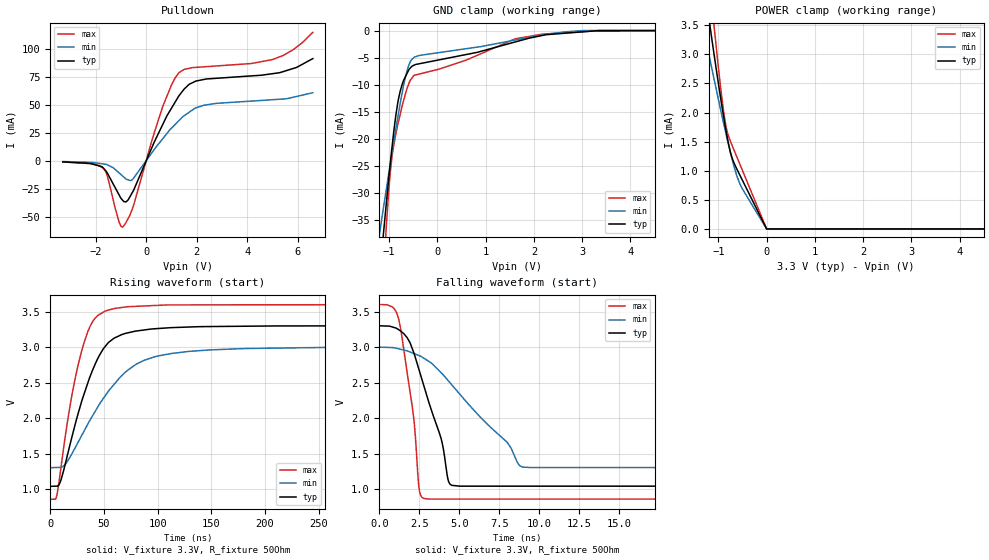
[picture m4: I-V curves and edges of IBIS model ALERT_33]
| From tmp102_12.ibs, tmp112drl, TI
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|   ALERT_33   3.3V digital open-drain Model
[Model] ALERT_33
Model_type   Open_drain
| Signals   ALERT(3)
Polarity   Non-Inverting
Enable   Active-Low
Vmeas = 1.65
Vref = 1.65
Cref = 15pF
Rref = 50
|   typ   min   max
|   (nom PVT)   (Fast PVT)   (slow PVT)
|   output low
|C_comp   1.4655810e-10   5.2129330e-11  1.1989730e-10
| Where   nom PVT is  Nominal Process, 3.3V, -40C
|   Fast PVT is Strong Process, 3.6V, 125C
|   Slow PVT is Weak Process, 3.0V, 27C
|   output high
C_comp   1.8565580e-12  1.4984630e-12  2.4264050e-12
| Where   nom PVT is  Nominal Process, 1.5V, 27C
|   Fast PVT is Strong Process, 1.6V, -40C
|   Slow PVT is Weak Process, 1.4V, 125C
[Voltage Range]   3.3   3   3.6
[Temperature Range]   27   125   -40
|Ambient Temperature   27   125   -40
[Pullup Reference]   3.3   3   3.6
[Pulldown Reference]   0   0   0
[Power Clamp Reference]   3.3   3   3.6
[GND Clamp Reference]   0   0   0
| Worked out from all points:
|   slope of the pulldown table from 0 to 0.495 V, typ, clamps not added: 19.8 ohm
|   POWER clamp passes 1 mA (typ) near -0.60 V on its own axis
|   falling waveform, V_fixture 3.3V, R_fixture 50Ohm: 20-80 % time 1.8ns typ, 4.29ns min, 878ps max; typ from 3.3 V to 1.04 V
|   rising waveform, V_fixture 3.3V, R_fixture 50Ohm: 20-80 % time 28.3ns typ, 45.8ns min, 20.4ns max; typ from 1.04 V to 3.3 V
[Pulldown]
|   Voltage   I(typ)   I(min)   I(max)
-3.3V     -1.098mA   -766.7uA   -1.108mA
-1.681V   -7.048mA   -2.977mA   -7.001mA
-1.529V   -11.45mA   -3.762mA   -14.26mA
-1.081V   -30.2mA    -10.78mA   -54.17mA
-934mV    -35.29mA   -13.71mA   -59.33mA
-794.1mV  -36.71mA   -16.5mA    -54.94mA
-537.4mV  -27.98mA   -16.79mA   -42.31mA
640.8mV   31.68mA    19.25mA    47.51mA
1.291V    57.8mA     35.63mA    78.35mA
1.965V    71.04mA    47.11mA    83.23mA
4.993V    77.6mA     54.39mA    90.18mA
6.59V     91.08mA    60.65mA    114.5mA
[GND Clamp]
|   Voltage   I(typ)   I(min)   I(max)
-3.3V     -260mA     -167.9mA   -426mA
-1.195V   -44.81mA   -37.4mA    -57.12mA
-1.112V   -37.03mA   -32.47mA   -44.03mA
-1.059V   -32.1mA    -29.45mA   -36.35mA
-995.2mV  -26.28mA   -25.75mA   -28.25mA
-943.3mV  -21.87mA   -22.76mA   -23.58mA
-809.8mV  -12.82mA   -15.55mA   -17.02mA
-646.4mV  -8.256mA   -8.026mA   -11.23mA
-477.1mV  -6.39mA    -4.916mA   -8.286mA
1.607V    -2.131mA   -1.766mA   -1.559mA
2.19V     -885.4uA   -771.3uA   -656.3uA
6.59V     0A         0A         0A
[POWER Clamp]
|   Voltage   I(typ)   I(min)   I(max)
-3.3V     16.57mA    11.82mA    23.43mA
-1.357V   4.569mA    3.65mA     5.784mA
-1.285V   4.144mA    3.363mA    5.158mA
-1.164V   3.432mA    2.873mA    4.115mA
-1.081V   2.96mA     2.548mA    3.431mA
-978.5mV  2.391mA    2.147mA    2.623mA
-897mV    1.963mA    1.838mA    2.059mA
-814.5mV  1.569mA    1.536mA    1.663mA
-714.3mV  1.217mA    1.196mA    1.434mA
-560.7mV  934.2uA    788.4uA    1.125mA
986.3uV   -1.645uA   -1.353uA   -1.987uA
6.59V     -1.645uA   -1.353uA   -1.987uA
[Ramp]
R_load = 50
|   typ   min   max
dV/dt_r   1.35577/2.83454e-008   1.01811/4.58016e-008   1.64544/2.04062e-008
dV/dt_f   1.35577/1.79966e-009   1.01811/4.27976e-009   1.64544/8.77153e-010
[Falling Waveform]
V_fixture = 3.3V
V_fixture_min = 3V
V_fixture_max = 3.6V
R_fixture = 50Ohm
C_fixture = 0F
|   Time   V(typ)   V(min)   V(max)
0s        3.3V       3V         3.6V
1.193ns   3.247V     2.977V     3.403V
2.141ns   2.926V     2.911V     2.01V
2.502ns   2.663V     2.879V     978.7mV
3.175ns   2.166V     2.787V     861.3mV
3.867ns   1.707V     2.638V     861.2mV
4.412ns   1.072V     2.5V       861.2mV
8.761ns   1.043V     1.335V     861.2mV
9.434ns   1.043V     1.305V     861.2mV
418.7ns   1.04V      1.303V     857.6mV
[Rising Waveform]
V_fixture = 3.3V
V_fixture_min = 3V
V_fixture_max = 3.6V
R_fixture = 50Ohm
C_fixture = 0F
|   Time   V(typ)   V(min)   V(max)
0s        1.04V      1.303V     857.6mV
6.21ns    1.043V     1.306V     916.9mV
9.86ns    1.124V     1.307V     1.294V
18.85ns   1.656V     1.464V     2.213V
29.96ns   2.271V     1.776V     2.985V
39.1ns    2.664V     2.026V     3.35V
50.48ns   2.996V     2.3V       3.503V
79.27ns   3.225V     2.752V     3.574V
112.9ns   3.274V     2.91V      3.594V
418.7ns   3.3V       3V         3.6V
